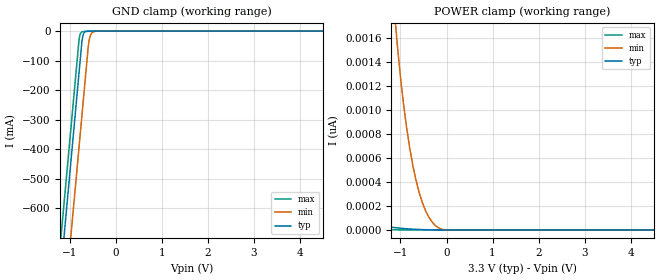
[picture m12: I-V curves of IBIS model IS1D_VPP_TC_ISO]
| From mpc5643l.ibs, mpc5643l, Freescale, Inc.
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| *** New cell (Generated with 5.14beta1 (Sep 20 2010 13:23:23))
[Model]   IS1D_VPP_TC_ISO
Model_type Input
Polarity   Non-Inverting
Enable   Active-Low
| CAP_THRESHOLD on pad vpp is "CMOS" :
| Rising=10.0% of VDDE1   Falling=90.0% of VDDE1
| C_comp min and max val. don't necessarily correlate with the min and max pvt
| but are the smallest and greatest pad capacitance found.
| var   typ   min   max
C_comp   15.69334pF  13.87408pF  18.06773pF
Vinl = 800.0mV | Dummy value overriden by next lines
Vinh = 2.0V | Dummy value overriden by next lines
[Model Spec]
| TIME_THRESHOLD on pin ipp_ind is "CORE" :
| Rising=40.0% of VDD   Falling=60.0% of VDD
Vinl 1.31250V 1.23650V 1.37750V
Vinh 1.94450V 1.73950V 2.18250V
| variable   typ   min   max
[Temperature Range] 25.0 150.0 -40.0
| variable   typ   min   max
[Voltage Range] 3.3V 3.0V 3.6V
| variable   typ   min   max
[POWER Clamp Reference] 3.3V 3.0V 3.6V
| variable   typ   min   max
[GND Clamp Reference] 0V 0V 0V
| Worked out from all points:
|   GND clamp passes 1 mA (typ) near -0.63 V on its own axis
[POWER Clamp]
-3.3V     489.8pA    56.01nA    41.71pA
-2.85V    301.3pA    34.99nA    24.87pA
-2.35V    162.8pA    18.2nA     13.24pA
-1.14V    20.55pA    1.866nA    1.747pA
-1.07V    17.43pA    1.552nA    1.49pA
-1V       14.65pA    1.278nA    1.26pA
-870mV    10.33pA    864.3pA    899.3fA
-670mV    5.502pA    427.7pA    488.4fA
-530mV    3.198pA    234.5pA    288.1fA
-400mV    1.706pA    117.8pA    155.9fA
-130mV    163.6fA    9.73pA     15.4fA
6.6V      0A         0A         0A
[GND Clamp]
-3.3V     -4.397A    -4.648A    -4.285A
-1.28V    -963.2mA   -1.214A    -851.2mA
-1.08V    -623.2mA   -874.4mA   -511.2mA
-870mV    -266.2mA   -517.4mA   -154.2mA
-790mV    -130.2mA   -381.4mA   -22.31mA
-730mV    -30.79mA   -279.4mA   -2.705mA
-680mV    -4.706mA   -194.4mA   -1.252mA
-600mV    -388.3uA   -58.42mA   -569.6uA
-580mV    -251.9uA   -33.93mA   -463.2uA
-540mV    -130.9uA   -11.54mA   -295.3uA
-460mV    -48.71uA   -1.441mA   -96.98uA
6.6V      911.1pA    103.2nA    22.37pA
